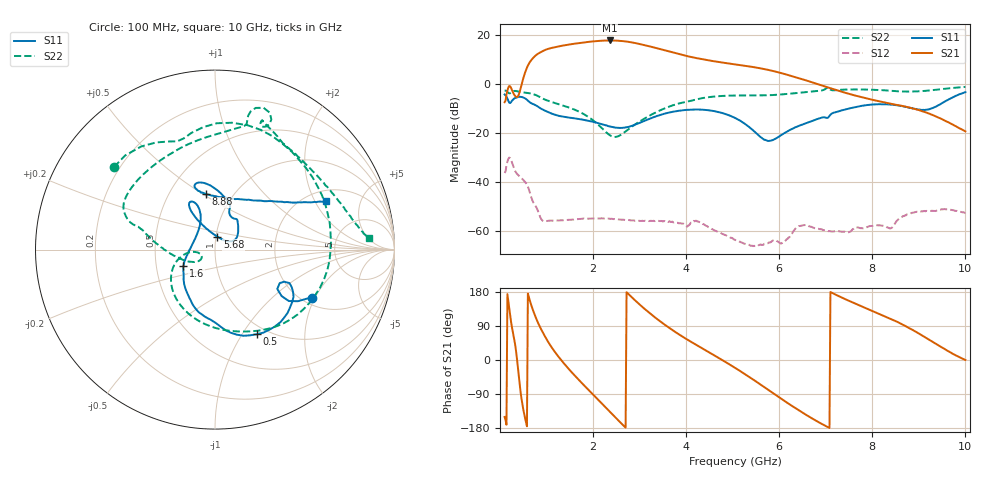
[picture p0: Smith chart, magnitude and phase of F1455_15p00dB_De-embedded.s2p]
! Integrated Device Technology
! Corporate Headquarters
! 6024 Silver Creek Valley Road
! San Jose, CA 95138  USA
! Phone:  1-408-284-8200
! Toll Free:  1-800-223-1366
! Webpage:  http://www.idt.com/
! Timing and RF Division
! 515 Groton Road, Suite 102
! Westford, MA 01886-6024
! Device:  F1455
! Description: 6-bit 0.5 dB Transmit Variable Gain Amplifier
! Frequency:  1400.0 -  2300.00 MHz
! Package:  6x6 mm Thin QFN Plastic Package: 28 pin
! State:  30
! Atten State:  15.0 dB
! Voltage:  +5.00 Volts
! Current:  217.658 mA
! Data:  The device was measured on a the F1455 evaluation board which has
!  individual transmission lines to the RF pins.  Data was collected
!  using a calibrated network analyzer.  The evaluation board was
!  de-embedded using a TRL calibration technique.
!  The reference plane is the edge of the package pin.
!  Pin  1 = CSb
!  Pin  2 = DATA
!  Pin  3 = CLK
!  Pin  4 = RSET
!  Pin  5 = GND
!  Pin  6 = RFIN  = Port 1
!  Pin  7 = GND
!  Pin  8 = NC
!  Pin  9 = NC
!  Pin 10 = NC
!  Pin 11 = NC
!  Pin 12 = NC
!  Pin 13 = NC
!  Pin 14 = /STBY
!  Pin 15 = GND
!  Pin 16 = RFOUT  = Port 2
!  Pin 17 = GND
!  Pin 18 = NC
!  Pin 19 = NC
!  Pin 20 = NC
!  Pin 21 = GND
!  Pin 22 = NC
!  Pin 23 = GND
!  Pin 24 = NC
!  Pin 25 = NC
!  Pin 26 = NC
!  Pin 27 = GND
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# GHz S dB R 50
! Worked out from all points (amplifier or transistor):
!   496 points, 100 MHz to 10 GHz, reference 50 ohm
!   highest |S21| = 17.6 dB at 2.36 GHz (marker M1)
!   |S21| within 3 dB of that: 1.119 GHz to 3.338 GHz (2.219 GHz wide, 99.5 % of centre)
!   unconditionally stable (mu >= 1): start of sweep to end of sweep
!   at 1.74 GHz: K = 36.89, MAG = 17.1 dB, |S12| = -55.0 dB
!   at 5.06 GHz: K = 194.66, MAG = 9.8 dB, |S12| = -63.6 dB
!   at 10 GHz: K = 271.51, MAG = -10.8 dB, |S12| = -52.4 dB
!   S11 on the Smith chart (normalised r, x): 100 MHz: 2.25, -1.91; 500 MHz: 0.89, -1.16; 1.6 GHz: 0.69, -0.13; 5.68 GHz: 1.02, +0.15; 8.88 GHz: 0.75, +0.52; 10 GHz: 2.47, +2.46
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0.1  -4.36 -26.4  -7.50 -150.3  -36.28 46.1  -2.77 140.7
0.24  -7.43 -24.9  -1.72 99.6  -31.04 -63.2  -3.56 101.4
0.38  -5.41 -41.0  -5.25 -13.3  -36.91 -115.3  -3.10 57.4
0.5  -5.58 -63.7  2.14 -129.7  -39.10 -153.4  -3.50 27.0
0.68  -7.97 -91.6  9.80 142.0  -46.57 143.6  -4.02 -15.1
0.8  -9.09 -107.0  12.01 103.1  -50.97 125.2  -4.83 -42.5
0.94  -10.69 -121.3  13.49 68.3  -55.96 123.6  -6.21 -68.8
1.26  -13.03 -141.7  15.21 8.4  -55.63 95.4  -8.28 -112.8
1.6  -14.04 -152.6  16.31 -40.2  -55.17 64.5  -10.50 -145.2
1.76  -14.52 -156.9  16.72 -60.9  -54.92 52.7  -11.91 -156.9
2.06  -15.76 -166.8  17.36 -98.6  -54.82 34.1  -15.79 -172.2
2.36  -17.36 175.3  17.63 -136.4  -54.92 18.7  -20.91 -166.8
2.76  -17.56 138.3  17.07 174.1  -55.47 2.0  -18.52 -146.1
3.06  -15.43 118.7  15.94 140.0  -55.71 -7.1  -14.65 -161.7
3.4  -12.96 111.7  14.32 105.9  -55.74 -17.7  -11.19 -179.3
4.08  -10.54 115.7  11.01 49.8  -57.14 -32.0  -7.01 163.4
5.06  -13.97 120.8  7.89 -21.4  -63.59 -74.5  -4.77 148.1
5.68  -22.78 79.8  5.98 -71.6  -65.11 -55.4  -4.70 123.0
6.7  -15.21 42.2  0.64 -153.7  -58.24 -130.7  -3.14 78.4
8.36  -8.41 107.0  -8.04 110.1  -58.71 150.4  -2.79 62.2
8.88  -10.11 99.1  -10.11 78.5  -52.39 140.3  -3.15 41.7
10  -3.43 23.8  -19.36 0.1  -52.45 61.1  -1.28 4.4
